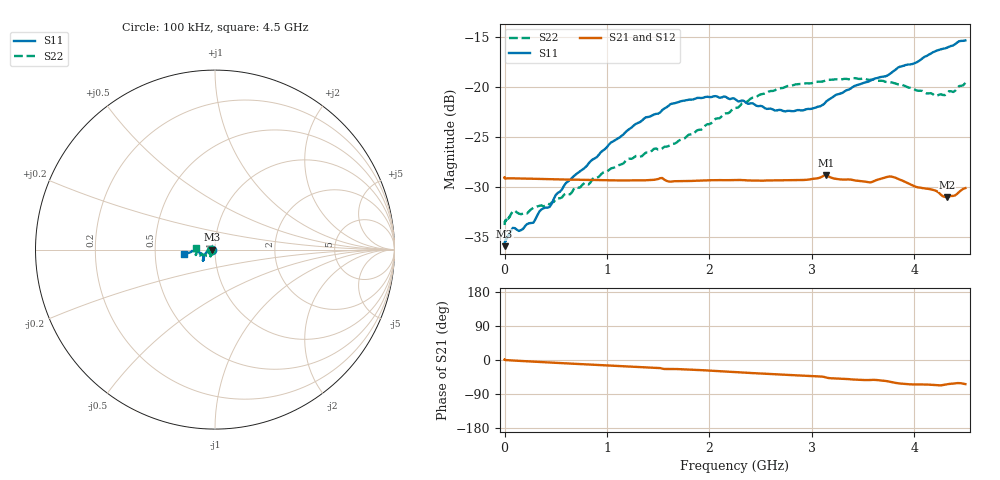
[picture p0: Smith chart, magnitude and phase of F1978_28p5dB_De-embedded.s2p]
! Integrated Device Technology
! Corporate Headquarters
! 6024 Silver Creek Valley Road
! San Jose, CA 95138  USA
! Phone:  1-408-284-8200
! Toll Free:  1-800-223-1366
! Webpage:  http://www.idt.com/
! Timing and RF Division
! 515 Groton Road, Suite 102
! Westford, MA 01886-6024
! Device:  F1978
! Description: 6-bit, 75 ohm, 0.5 dB Digital Step Attenuator
! Frequency:  5.0 MHz -  3.00 GHz
! Package:  4x4 mm QFN Plastic Package: 20 pin
! Ports:  2 RF, 11 DC
!  Pin  1  = D5 (16 dB)
!  Pin  2  = RF1  =  Port 1
!  Pin  3  = Serial Data In (DATA)
!  Pin  4  = Serial Clock (CLK)
!  Pin  5  = Serial Latch Enable (LE)
!  Pin  6  = VDD
!  Pin  7  = NC
!  Pin  8  = NC
!  Pin  9  = NC
!  Pin 10  = GND
!  Pin 11  = GND
!  Pin 12  = NC
!  Pin 13  = VMODE
!  Pin 14  = RF2  =  Port 2
!  Pin 15  = D4 (8 dB)
!  Pin 16  = D3 (4 dB)
!  Pin 17  = D2 (2 dB)
!  Pin 18  = NC
!  Pin 19  = D1 (1 dB)
!  Pin 20  = D0 (0.5 dB)
! State:  57
! Atten State:  28.5 dB
! Voltage:  +3.30 Volts
! Current:  0.564 mA
! Data:  The device was measured on a F1975 evaluation board which has
!  individual transmission lines to the RF pins.  Data was collected
!  using a calibrated network analyzer.  The evaluation board was
!  de-embedded using Automatic Fixture Removal (AFR).
!  The reference plane is the edge of the package pin.
! Misc:
!  Action Tracker AT0416
! Date Measured:  2018-02-08
! Date:  2018-03-26  MJV
! Note:
!  Integrated Device Technology supplies this data as a sample of measured
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# GHz S dB R 75
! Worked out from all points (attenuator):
!   291 points, 100 kHz to 4.5 GHz, reference 75 ohm
!   highest |S21| = -28.83 dB at 3.14 GHz (marker M1); lowest = -31.0 dB at 4.32 GHz (marker M2)
!   lowest |S11| = -36.0 dB at 100 kHz (marker M3), VSWR 1.03, Z = 72.6 + j0.00127 ohm
!   |S11| at or under -10 dB: start of sweep to end of sweep
!   |S22| runs from -33.8 to -19.1 dB; largest |S21 - S12| = 0.0002
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0.0001  -35.95 180.0  -29.07 1.2  -29.10 1.2  -33.83 -178.9
0.007  -35.39 -178.4  -29.13 0.2  -29.14 0.2  -33.44 -177.3
0.08  -34.12 -176.6  -29.15 -1.3  -29.14 -1.3  -32.44 -169.5
0.14  -34.42 -175.8  -29.15 -2.2  -29.15 -2.2  -32.69 -161.1
0.28  -33.61 179.3  -29.19 -4.3  -29.19 -4.3  -32.11 -151.9
0.34  -32.47 178.0  -29.21 -5.2  -29.21 -5.2  -31.91 -146.9
0.44  -32.01 -179.9  -29.23 -6.6  -29.22 -6.6  -31.76 -138.8
0.6  -29.61 -176.4  -29.27 -8.9  -29.26 -8.9  -30.66 -133.0
0.76  -28.27 -169.6  -29.29 -11.1  -29.30 -11.1  -29.79 -129.0
1.28  -23.70 -153.2  -29.35 -17.9  -29.35 -17.9  -26.91 -124.7
1.52  -22.52 -145.1  -29.13 -21.4  -29.12 -21.4  -26.26 -131.2
1.62  -21.70 -143.3  -29.48 -23.4  -29.48 -23.4  -25.80 -134.6
1.88  -21.08 -139.3  -29.38 -26.2  -29.38 -26.2  -24.32 -147.1
2.26  -21.27 -138.2  -29.32 -32.0  -29.32 -32.0  -22.08 -158.0
2.64  -22.34 -147.5  -29.35 -37.5  -29.35 -37.5  -20.31 -159.4
3.02  -22.10 -164.0  -29.18 -42.6  -29.18 -42.6  -19.53 -160.0
3.14  -21.44 -166.7  -28.83 -46.2  -28.83 -46.2  -19.30 -160.5
3.56  -19.41 -177.2  -29.54 -52.9  -29.54 -52.9  -19.28 -165.9
3.76  -18.69 -175.9  -28.96 -57.2  -28.96 -57.2  -19.52 -169.6
4.2  -16.42 -172.7  -30.35 -66.1  -30.35 -66.2  -20.85 178.9
4.32  -16.04 -172.4  -31.03 -64.1  -31.03 -64.1  -20.62 176.6
4.5  -15.31 -172.3  -30.13 -63.6  -30.12 -63.6  -19.56 173.9
